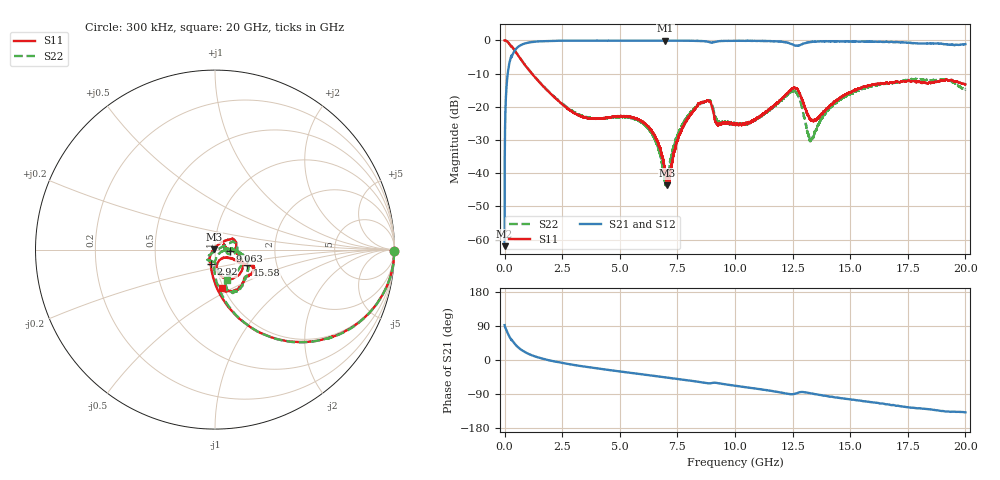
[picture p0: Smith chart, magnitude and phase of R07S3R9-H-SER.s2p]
!{R07S3R9}
!Johanson Technology Inc.
!www.johansontechnology.com
!Test Board Conditions:
!Substrate Type  RO4350B
!Substrate Thickness  10 mil
!Substrate Dk  3.66
!TL Type: GCPW
!TL Trace Width  21 mil
!TL Gap  20 mil
!Electrode orientation  Horizontal
!DUT TOPOLOGY	SERIES
!Mounting Pad LxW  16x21 mil
! Created Sat Feb  6 11:32:35 2021
# hz S ma R 50
! 2 Port Network Data from SP1.SP block
! freq  magS11  angS11  magS21  angS21  magS12  angS12  magS22  angS22
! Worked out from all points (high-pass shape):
!   20001 points, 300 kHz to 20 GHz, reference 50 ohm
!   highest |S21| = -0.03 dB at 6.974 GHz (marker M1); lowest = -62.0 dB at 300 kHz (marker M2)
!   |S21| within 3 dB of the highest: 442.5 MHz to end of sweep
!   lowest |S11| = -43.6 dB at 7.055 GHz (marker M3), VSWR 1.01, Z = 49.4 + j0.24 ohm
!   |S11| at or under -10 dB: 1.188 GHz to end of sweep
!   |S22| runs from -43.6 to 0.0 dB; largest |S21 - S12| = 0.013
!   S11 on the Smith chart (normalised r, x): 300 kHz: open; 2.92 GHz: 0.94, -0.16; 9.063 GHz: 1.18, -0.02; 15.58 GHz: 1.41, -0.26; 20 GHz: 0.98, -0.44
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300000  0.9988 -0.4  0.0007989 92.0  0.0007137 91.8  1 -0.5
1.153e8  0.9599 -16.6  0.2746 73.7  0.2749 73.6  0.9605 -16.6
3.363e8  0.794 -38.7  0.6012 50.9  0.6019 50.9  0.7936 -38.7
1.0983e9  0.3441 -75.6  0.9358 14.6  0.9368 14.5  0.347 -74.9
2.9203e9  0.08553 -106.2  0.9925 -12.2  0.9929 -12.3  0.08777 -94.0
3.3343e9  0.07196 -109.8  0.9931 -16.2  0.9934 -16.2  0.07419 -96.4
5.7423e9  0.06588 -118.9  0.9949 -36.1  0.9939 -36.0  0.06375 -132.2
6.6673e9  0.02868 -135.6  0.9955 -43.3  0.9954 -43.4  0.02445 -127.6
6.9743e9  0.0103 -170.3  0.9967 -45.9  0.9955 -45.8  0.007131 -78.9
7.0553e9  0.006571 158.3  0.9936 -46.5  0.9958 -46.5  0.008135 -31.2
7.3923e9  0.02277 64.7  0.9931 -49.1  0.9941 -49.2  0.02892 16.9
7.8793e9  0.06016 46.0  0.99 -53.1  0.9905 -53.1  0.06615 23.9
8.7453e9  0.1218 24.4  0.9676 -60.7  0.9663 -60.7  0.1204 14.8
9.0633e9  0.08298 -5.7  0.9368 -60.2  0.936 -60.2  0.09226 -17.3
9.2463e9  0.05376 15.9  0.9693 -60.8  0.9687 -60.9  0.05857 -7.5
1.00003e10  0.05502 26.0  0.9891 -67.9  0.9884 -68.0  0.05443 5.3
1.25733e10  0.1955 -46.9  0.8448 -89.4  0.8464 -89.6  0.1747 -46.6
1.33343e10  0.06293 -63.4  0.9523 -88.4  0.9525 -88.5  0.03322 -34.6
1.41853e10  0.1098 -28.7  0.97 -96.7  0.9697 -96.9  0.1015 -1.3
1.55753e10  0.2004 -25.7  0.9627 -108.7  0.9618 -108.6  0.1889 -18.5
1.66673e10  0.2259 -23.5  0.9404 -117.2  0.9465 -117.6  0.2266 -39.2
2e10  0.2184 -80.0  0.8798 -138.0  0.8745 -137.9  0.1831 -68.3
